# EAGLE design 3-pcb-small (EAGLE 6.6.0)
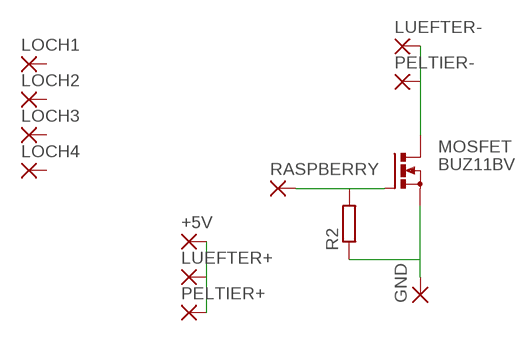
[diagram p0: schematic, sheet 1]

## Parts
+5V  2,54/1,0  [2,54/1,0]
GND  2,54/1,0  [2,54/1,0]
LOCH1  2,54/1,0  [2,54/1,0]
LOCH2  2,54/1,0  [2,54/1,0]
LOCH3  2,54/1,0  [2,54/1,0]
LOCH4  2,54/1,0  [2,54/1,0]
LUEFTER+  2,54/1,0  [2,54/1,0]
LUEFTER-  2,54/1,0  [2,54/1,0]
MOSFET  BUZ11BV  [TO220BV]
PELTIER+  2,54/1,0  [2,54/1,0]
PELTIER-  2,54/1,0  [2,54/1,0]
R2  R-EU_0207/15  [0207/15]
RASPBERRY  2,54/1,0  [2,54/1,0]

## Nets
N$1: LUEFTER-.1(P) MOSFET.D PELTIER-.1(P)
N$2: MOSFET.G R2.2 RASPBERRY.1(P)
N$3: GND.1(P) MOSFET.S R2.1
N$4: +5V.1(P) LUEFTER+.1(P) PELTIER+.1(P)
Unconnected: LOCH1.1(P) LOCH2.1(P) LOCH3.1(P) LOCH4.1(P)

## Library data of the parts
+5V GND LOCH1-LOCH4 LUEFTER+ LUEFTER- PELTIER+ PELTIER- RASPBERRY = wirepad:2,54/1,0: THROUGH-HOLE PAD
MOSFET = transistor-power:BUZ11: N-CHANNEL MOS FET
R2 = resistor:R-EU_: RESISTOR, European symbol

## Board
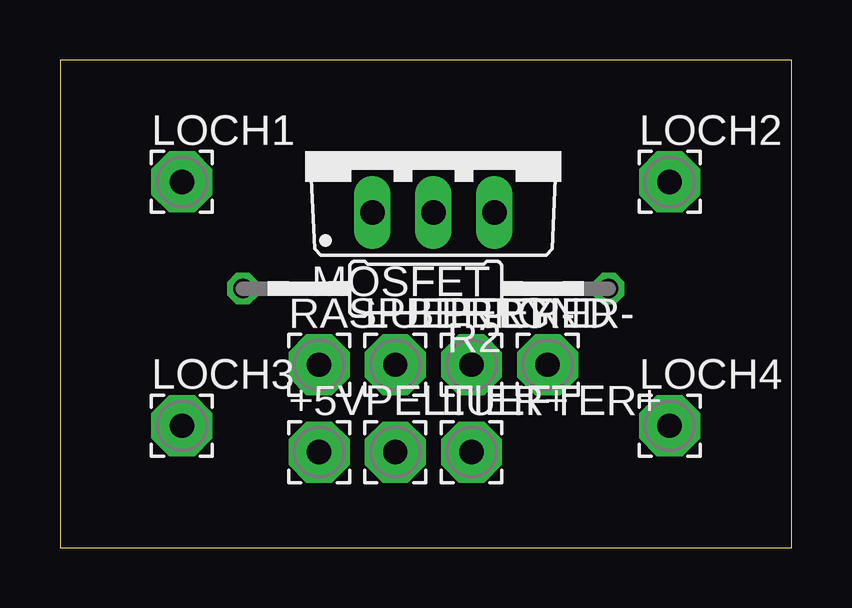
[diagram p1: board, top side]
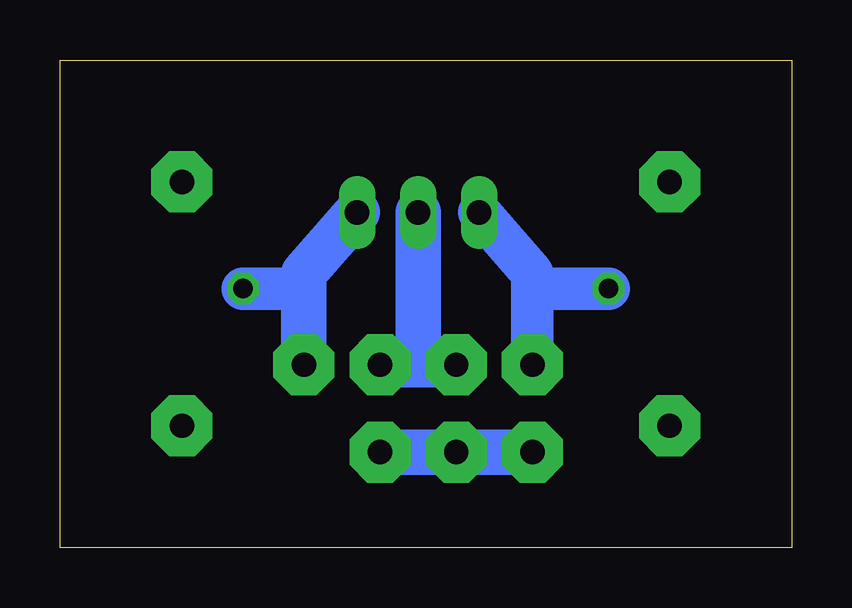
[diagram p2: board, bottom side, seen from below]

Size 30.48 x 20.32 mm. Coordinates in mm from the lower left corner, seen from the top.
Outline: 0,0 30.48,0 30.48,20.32 0,20.32 0,0
Copper layers (1*16): Top 0.035mm / dielectric 1.5mm / Bottom 0.035mm
Design rules "default": minimum track width 10mil, minimum drill 24mil, track to track 8mil, track to pad 8mil, pad to pad 8mil, via to via 8mil, smd to smd 8mil, copper to edge 40mil, drill to drill 8mil, minimum pad ring 10mil, minimum via ring 8mil, stop-mask expansion 4mil, vias tented up to drill 0mil, thermal gap 10mil

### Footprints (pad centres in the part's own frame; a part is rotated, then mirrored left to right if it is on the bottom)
2,54/1,0 = drill 1.016 pad 2.54 octagon: 1 0,0
TO220BV = drill 1.016 long: D 0,-2.54; G -2.54,-2.54; S 2.54,-2.54
0207/15 = drill 0.813 octagon: 1 -7.62,0; 2 7.62,0

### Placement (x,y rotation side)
+5V  10.79,3.98 0 top
GND  20.32,7.62 0 top
LOCH1  5.08,15.24 0 top
LOCH2  25.4,15.24 0 top
LOCH3  5.08,5.08 0 top
LOCH4  25.4,5.08 0 top
LUEFTER+  17.14,3.98 0 top
LUEFTER-  13.97,7.62 0 top
MOSFET  15.56,16.51 0 top
PELTIER+  13.97,3.98 0 top
PELTIER-  17.14,7.62 0 top
R2  15.24,10.79 180 top
RASPBERRY  10.79,7.62 0 top

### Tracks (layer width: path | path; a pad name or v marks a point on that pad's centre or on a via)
N$1
  Bottom 1.905: LUEFTER-.1 15.56,7.62 | 15.56,7.62 PELTIER-.1 | MOSFET.D 15.56,7.62
N$2
  Bottom 1.778: MOSFET.G 10.79,11.43 10.79,10.79 | 10.79,10.79 RASPBERRY.1 | R2.2 10.79,10.79
N$3
  Bottom 1.778: R2.1 20.32,10.79
  Bottom 1.905: MOSFET.S 20.32,11.43 20.32,10.79 GND.1
N$4
  Bottom 1.905: +5V.1 PELTIER+.1 LUEFTER+.1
